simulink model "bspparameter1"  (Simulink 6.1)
settings: Solver=ode45  SolverMode=SingleTasking  StartTime=0.0  StopTime=500.0  FixedStep=0.01  RelTol=1e-3
PreLoadFcn:
  | bspparameter_ini
InitFcn:
  | bspparameter_ini
StopFcn:
  | bspparameter1_plot
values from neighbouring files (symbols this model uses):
  Konst = 1.15    [bspparameter_ini.m]    (also in bsp_parameter_ini.m)
  verst = 10    [bspparameter_ini.m]    (also in bsp_parameter_ini.m)
libraries: simulink x1

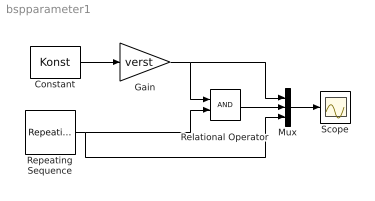
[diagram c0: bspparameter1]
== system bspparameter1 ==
  Constant : Constant  Value=Konst
  Gain : Gain  Gain=verst
  Mux : Mux  Inputs=3
  Relational Operator : RelationalOperator
  Repeating Sequence : simulink/Sources/Repeating Sequence  rep_seq_t=zeit  rep_seq_y=wiederhol
  Scope : Scope
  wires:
  Relational Operator/1 -> Mux/2
  Repeating Sequence/1 -> Relational Operator/2, Mux/3
  Constant/1 -> Gain/1
  Gain/1 -> Relational Operator/1, Mux/1
  Mux/1 -> Scope/1
